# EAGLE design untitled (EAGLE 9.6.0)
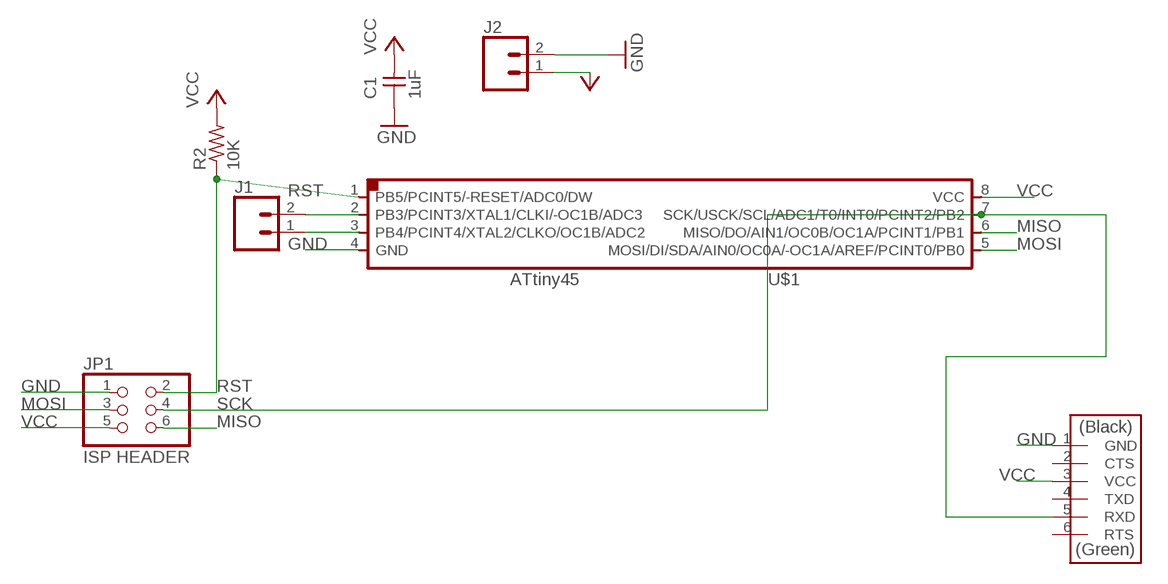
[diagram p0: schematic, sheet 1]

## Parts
C1  1uF  CAP-UNPOLARIZEDFAB  [C1206FAB]
J1  CONN_02  [1X02]
J2  CONN_02  [1X02]
JP1  ISP HEADER  PINHD-2X3-SMD  [2X03SMD]
R2  10K  RES-US1206FAB  [R1206FAB]
U$1  ATTINY45SI  [SOIC8]
U$2  FTDI-SMD-HEADER  [1X06SMD]

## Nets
GND: C1.1 J2.2 JP1.1 U$1.4(GND) U$2.1(GND)
MISO: JP1.6 U$1.6(MISO/DO/AIN1/OC0B/OC1A/PCINT1/PB1)
MOSI: JP1.3 U$1.5(MOSI/DI/SDA/AIN0/OC0A/-OC1A/AREF/PCINT0/PB0)
N$1: J1.2 U$1.2(PB3/PCINT3/XTAL1/CLKI/-OC1B/ADC3)
N$2: J1.1 U$1.3(PB4/PCINT4/XTAL2/CLKO/OC1B/ADC2)
RST: JP1.2 R2.1 U$1.1(PB5/PCINT5/-RESET/ADC0/DW)
SCK: JP1.4 U$1.7(SCK/USCK/SCL/ADC1/T0/INT0/PCINT2/PB2) U$2.5(RXD)
VCC: C1.2 J2.1 JP1.5 R2.2 U$1.8(VCC) U$2.3(VCC)
Unconnected: U$2.2(CTS) U$2.4(TXD) U$2.6(RTS)

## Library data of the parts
C1 = fab:CAP-UNPOLARIZED
J1 J2 = SparkFun-Connectors:CONN_02: Multi connection point. Often used as Generic Header-pin footprint for 0.1 inch spaced/style header connections
JP1 = fab:PINHD-2X3-SMD: PIN HEADER
R2 = fab:RES-US: Resistor (US Symbol)
U$1 = fab:ATTINY45
U$2 = fab:FTDI-SMD-HEADER

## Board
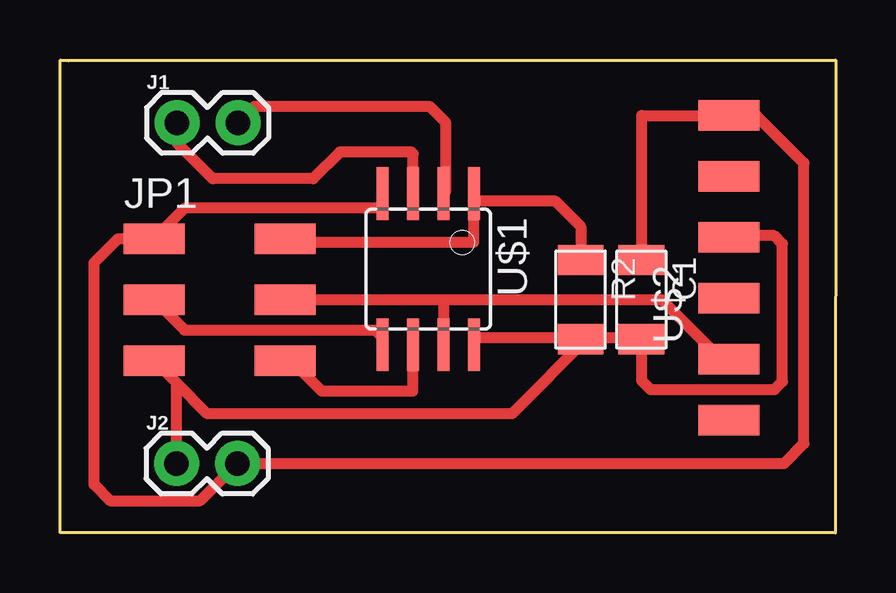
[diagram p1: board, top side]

Size 32.34 x 19.73 mm. Coordinates in mm from the lower left corner, seen from the top.
Outline: 0.36,19.68 0.01,19.72
Outline: 0.01,19.72 32.34,19.73 32.33,0 0,0.01 0.01,19.72
Copper layers (1*16): Top 0.035mm / dielectric 1.5mm / Bottom 0.035mm
Design rules "default *": minimum track width 18mil, minimum drill 0.35mm, track to track 16mil, track to pad 16mil, pad to pad 16mil, via to via 6mil, smd to smd 16mil, copper to edge 40mil, drill to drill 6mil, minimum pad ring 10mil, minimum via ring 8mil, stop-mask expansion 4mil, vias tented up to drill 0mil, thermal gap 10mil

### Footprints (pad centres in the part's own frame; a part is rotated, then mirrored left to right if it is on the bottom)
C1206FAB = smd 1.27 x 1.905: 1 -1.651,0; 2 1.651,0
1X02 = drill 1.016 pad 1.88: 1 0,0; 2 2.54,0
2X03SMD = smd 2.54 x 1.27: 1 -2.54,2.54; 2 2.92,2.54; 3 -2.54,0; 4 2.92,0; 5 -2.54,-2.54; 6 2.92,-2.54
R1206FAB = smd 1.27 x 1.905: 1 -1.651,0; 2 1.651,0
SOIC8 = smd 0.5 x 2.2: 1 -1.905,-3.154; 2 -0.645,-3.154; 3 0.625,-3.154; 4 1.895,-3.154; 5 1.905,3.154; 6 0.635,3.154; 7 -0.635,3.154; 8 -1.905,3.154
1X06SMD = smd 2.54 x 1.27: 1 0,6.35; 2 0,3.81; 3 0,1.27; 4 0,-1.27; 5 0,-3.81; 6 0,-6.35

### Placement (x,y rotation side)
C1  24.24,9.73 270 top
J1  4.88,17.11 0 top
J2  4.86,2.9 0 top
JP1  6.46,9.73 0 top
R2  21.7,9.73 270 top
U$1  15.35,11 180 top
U$2  27.88,11.06 0 top

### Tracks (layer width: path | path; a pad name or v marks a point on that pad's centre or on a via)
GND
  Top 0.457: 13.45,13.54 13.45,13.86 U$1.4 13.45,13.54 | 13.45,13.54 5.19,13.54 JP1.1 2.42,12.27 1.42,11.27 1.42,2.03 2.12,1.33 5.82,1.33 J2.2 30.19,2.9 31.02,3.73 31.02,15.43 29.03,17.41 U$2.1 24.24,17.41 C1.1 24.19,11.39
MISO
  Top 0.457: U$1.6 14.72,5.92 10.91,5.92 9.64,7.19 JP1.6
MOSI
  Top 0.457: JP1.3 5.19,8.46 13.13,8.46 13.45,8.15 U$1.5
N$1
  Top 0.457: J1.2 8.11,17.8 15.4,17.8 16.09,17.11 16.09,14.25 U$1.2
N$2
  Top 0.457: U$1.3 14.73,15.81 14.64,15.89 11.67,15.89 10.55,14.78 6.37,14.78 4.88,16.27 J1.1
RST
  Top 0.457: 17.26,13.86 U$1.1 | JP1.2 9.53,12.13 17.26,12.13 17.26,13.86 | 17.26,13.86 20.63,13.86 21.72,12.78 21.72,11.4 R2.1
SCK
  Top 0.457: 15.99,9.73 U$1.7 | JP1.4 15.99,9.73 | 27.6,7.25 U$2.5 27.56,7.25 25.08,9.73 15.99,9.73
VCC
  Top 0.457: 21.7,8.15 22.02,8.15 | 21.7,8.15 17.26,8.15 U$1.8 | 22.02,8.15 24.24,8.15 C1.2 24.24,6.36 24.62,5.98 29.79,5.98 30.12,6.32 30.12,12.06 29.78,12.4 27.95,12.4 U$2.3 | 21.7,8.15 R2.2 | 4.86,6.26 6.15,4.97 18.85,4.97 22.02,8.15 | JP1.5 4.67,6.45 4.86,6.26 | J2.1 4.86,6.26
